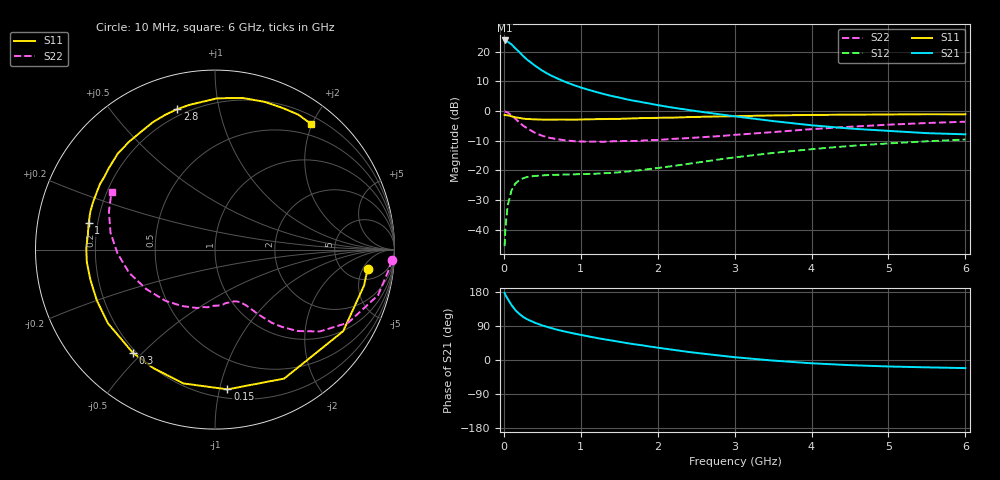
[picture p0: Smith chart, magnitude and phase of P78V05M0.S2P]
! SIEMENS Small Signal Semiconductors
! BFP196
! Si NPN RF Bipolar Junction Transistor in SOT143
! VCE = 8 V  IC = 5 mA
! Common Emitter S-Parameters:  May  1996
# GHz  S  MA  R  50
!  f  S11  S21  S12  S22
! GHz  MAG  ANG  MAG  ANG  MAG  ANG  MAG  ANG
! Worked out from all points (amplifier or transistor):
!   36 points, 10 MHz to 6 GHz, reference 50 ohm
!   highest |S21| = 23.8 dB at 10 MHz (marker M1)
!   |S21| within 3 dB of that: start of sweep to 164.3 MHz
!   unconditionally stable (mu >= 1): 1.164 GHz to 3.258 GHz
!   at 250 MHz: K = 0.25, MSG = 20.6 dB, |S12| = -22.7 dB
!   at 1.4 GHz: K = 1.13, MAG = 10.8 dB, |S12| = -20.8 dB
!   at 6 GHz: K = 0.98, MSG = 0.9 dB, |S12| = -9.6 dB
!   S11 on the Smith chart (normalised r, x): 10 MHz: 8, -6; 150 MHz: 0.26, -1.06; 300 MHz: 0.19, -0.47; 1 GHz: 0.16, +0.10; 2.8 GHz: 0.17, +0.75; 6 GHz: 0.32, +1.99
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0.01  0.8574 -7.1  15.43 177.1  0.0053 87.9  0.9856 -3.4
0.02  0.8541 -13.6  15.12 172.0  0.0106 82.0  0.9758 -6.4
0.05  0.8464 -32.5  14.72 161.3  0.0258 72.1  0.9435 -15.6
0.1  0.8154 -61.8  13.24 145.1  0.0462 59.1  0.847 -28.7
0.15  0.7818 -84.9  11.37 131.6  0.06 48.1  0.7408 -38.0
0.2  0.7662 -103.3  9.881 121.8  0.0684 40.7  0.6462 -44.6
0.25  0.7441 -117.6  8.445 113.8  0.0735 34.9  0.5686 -49.2
0.3  0.7347 -128.6  7.386 107.8  0.0774 31.5  0.5158 -52.2
0.4  0.7242 -145.5  5.872 98.6  0.0806 26.3  0.4328 -56.3
0.5  0.7168 -156.8  4.777 91.2  0.0824 23.7  0.3824 -59.0
0.6  0.7142 -166.2  4.041 85.1  0.084 22.4  0.3531 -61.1
0.7  0.7175 -174.3  3.516 79.5  0.0844 21.5  0.3344 -63.2
0.8  0.7174 179.4  3.088 74.8  0.0854 21.5  0.3205 -65.5
1  0.7195 168.1  2.495 66.3  0.0865 23.0  0.3069 -70.4
1.1  0.7262 163.0  2.279 62.3  0.0871 24.1  0.3051 -73.1
1.6  0.7458 142.5  1.568 44.6  0.0956 31.1  0.3127 -87.7
2.2  0.7742 122.6  1.138 26.9  0.1186 38.5  0.3398 -106.7
2.8  0.8105 105.0  0.882 11.9  0.1531 39.4  0.3775 -127.3
3.5  0.8431 89.1  0.677 -1.5  0.1969 34.8  0.4417 -150.1
4.5  0.8683 71.4  0.507 -13.6  0.2582 24.0  0.5435 -177.7
5.5  0.8839 58.2  0.424 -19.4  0.3094 11.5  0.6279 160.3
6  0.8808 52.5  0.405 -21.4  0.3311 4.8  0.6605 150.8
